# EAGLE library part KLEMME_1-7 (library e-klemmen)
Klemme 7 Pol.
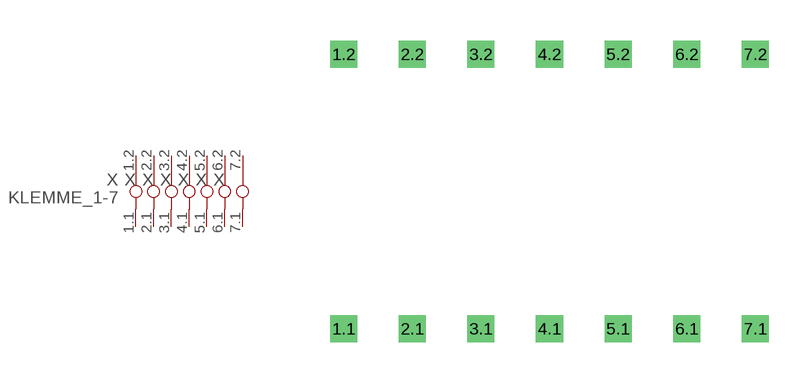
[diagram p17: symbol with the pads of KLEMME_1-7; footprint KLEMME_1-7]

Designator prefix X; gates 1=KLEMME_1-1 2=KLEMME_2 3=KLEMME_3 4=KLEMME_4 5=KLEMME_5 6=KLEMME_6 7=KLEMME_7

## KLEMME_1-7  [KLEMME_1-7]
1.1  1:1.1  pas
1.2  1:1.2  pas
2.1  2:2.1  pas
2.2  2:2.2  pas
3.1  3:3.1  pas
3.2  3:3.2  pas
4.1  4:4.1  pas
4.2  4:4.2  pas
5.1  5:5.1  pas
5.2  5:5.2  pas
6.1  6:6.1  pas
6.2  6:6.2  pas
7.1  7:7.1  pas
7.2  7:7.2  pas

## Footprint KLEMME_1-7 (pad centres in mm)
Dummy
drill 0.5 pad 1 square: 1.1 0,-12.7; 1.2 0,-2.54; 2.1 2.54,-12.7; 2.2 2.54,-2.54; 3.1 5.08,-12.7; 3.2 5.08,-2.54; 4.1 7.62,-12.7; 4.2 7.62,-2.54; 5.1 10.16,-12.7; 5.2 10.16,-2.54; 6.1 12.7,-12.7; 6.2 12.7,-2.54; 7.1 15.24,-12.7; 7.2 15.24,-2.54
